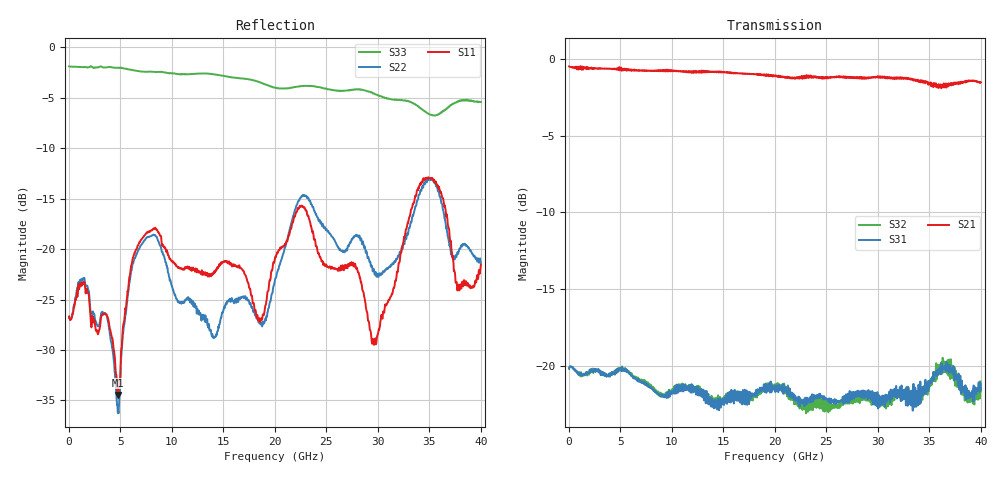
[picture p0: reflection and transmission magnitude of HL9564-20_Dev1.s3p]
! 10/7/2020 12:24:52 PM
! H:\PRODUCTION_DATA\TEMP_S3P.S3P
! CHANNEL.1
! TR.MEASUREMENT
! CORRECTED.DATA
# GHZ S RI R 50.0
! FREQ.GHZ  S11RE  S11IM  S12RE  S12IM  S13RE  S13IM
!  S21RE  S21IM  S22RE  S22IM  S23RE  S23IM
!  S31RE  S31IM  S32RE  S32IM  S33RE  S33IM
!; PortSelection: Port_123
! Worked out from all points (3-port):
!   1143 points, 35 MHz to 40.01 GHz, reference 50 ohm
!   strongest paths, dB at 35 MHz, 10.01 GHz, 20.02 GHz, 30.03 GHz, 40.01 GHz:
!     S21: -0.5, -0.8, -1.1, -1.2, -1.5
!     S31: -20.2, -21.8, -21.5, -22.8, -21.6
!     S32: -20.2, -21.8, -21.5, -22.6, -21.7
!   lowest |S11| = -34.5 dB at 4.76 GHz (marker M1), VSWR 1.04, Z = 48.2 - j0.513 ohm
!   |S11| at or under -10 dB: start of sweep to end of sweep
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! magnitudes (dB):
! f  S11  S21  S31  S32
! 35 MHz  -26.7  -0.5  -20.2  -20.2
! 3.57 GHz  -26.4  -0.6  -20.6  -20.6
! 4.76 GHz  -34.5  -0.7  -20.4  -20.4
! 7.595 GHz  -18.3  -0.7  -21.3  -21.3
! 14.07 GHz  -22.4  -0.8  -22.7  -22.5
! 20.02 GHz  -20.8  -1.1  -21.5  -21.5
! 22.79 GHz  -15.8  -1.1  -22.4  -22.6
! 29.71 GHz  -29.0  -1.2  -22.6  -22.5
! 35.03 GHz  -13.0  -1.6  -21.0  -21.0
! 40.01 GHz  -21.6  -1.5  -21.6  -21.7
